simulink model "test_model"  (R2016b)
settings: Solver=VariableStepAuto  StartTime=0.0  StopTime=runtime  RelTol=1e-3
InitFcn:
  | clear mex
  | delete test_model_sfun.mexw64
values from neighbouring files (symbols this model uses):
  Delta_T = cell(1,4)    [modelParameters.m]
  F_D = 0    [modelParameters.m]
  g = 9.81    [modelParameters.m]
  Gamma_H = cell(1,4)    [modelParameters.m]
  have_motor_transient = 1    [modelParameters.m]
  height_controlled_o = (((Rm*If        + (((omega0_o * 2 * Rm * Kv * Kq      * Kd + 1)^2) - 1)/(4* Rm*Kv^2*Kq      * Kd))/Vb)*(Pmax - Pmin) + Pmin)    [modelParameters.m]
  i_0 = cell(1,4)    [modelParameters.m]
  If = 0.3836    [modelParameters.m]
  J = diag([ 0.0130 0.0140 0.0285 ])    [modelParameters.m]
  J_L = m_L/12*diag([y_L^2+z_L^2,x_L^2+z_L^2,x_L^2+y_L^2])    [modelParameters.m]
  J_r = cell(1,4)    [modelParameters.m]
  Jreq = 4.2012e-05    [modelParameters.m]
  Jxx = 0.0130    (= 0.013)    [modelParameters.m]
  Jyy = 0.0140    (= 0.014)    [modelParameters.m]
  Jzz = 0.0285    [modelParameters.m]
  K_d = cell(1,4)    [modelParameters.m]
  K_E = cell(1,4)    [modelParameters.m]
  K_H = cell(1,4)    [modelParameters.m]
  K_Q = cell(1,4)    [modelParameters.m]
  K_T = cell(1,4)    [modelParameters.m]
  K_V = cell(1,4)    [modelParameters.m]
  Kd = 1.4852e-07    [modelParameters.m]
  Ki_mahony = 0.001    [modelParameters.m]
  Kp_mahony = 0.4    [modelParameters.m]
  Kq = 96.3422    [modelParameters.m]
  Kt = 1.2007e-05    [modelParameters.m]
  Kv = 96.3422    [modelParameters.m]
  m = 1.216    [modelParameters.m]
  m_L = 0    [modelParameters.m]
  omega0_o = sqrt((m*g)/(4*Kt))    [modelParameters.m]
  omega1_o = sqrt((m*g)/(4*Kt))    [modelParameters.m]
  omega2_o = sqrt((m*g)/(4*Kt))    [modelParameters.m]
  omega3_o = sqrt((m*g)/(4*Kt))    [modelParameters.m]
  omega_0 = cell(1,4)    [modelParameters.m]
  p0 = 0    [modelParameters.m]
  p_0 = cell(1,4)    [modelParameters.m]
  p_max = cell(1,4)    [modelParameters.m]
  phi0 = 0    [modelParameters.m]
  pitch_o = 0    [modelParameters.m]
  pitchrate_o = 0    [modelParameters.m]
  Pmax = 1    [modelParameters.m]
  Pmin = 0    [modelParameters.m]
  psi0 = 0    [modelParameters.m]
  q0 = 0    [modelParameters.m]
  Q_D = 0    [modelParameters.m]
  r0 = 0    [modelParameters.m]
  R_m = cell(1,4)    [modelParameters.m]
  r_oc = [ 0 ; 0 ; 0 ]    [modelParameters.m]
  r_oL = [0; 0; 0]    [modelParameters.m]
  rhx = 0.16    [modelParameters.m]
  rhy = 0.16    [modelParameters.m]
  rhz = 0.03    [modelParameters.m]
  Rm = 0.235    [modelParameters.m]
  roll_o = 0    [modelParameters.m]
  rollrate_o = 0    [modelParameters.m]
  Tc = 0.04    [modelParameters.m]
  theta0 = 0    [modelParameters.m]
  Tq = 0.005    [modelParameters.m]
  u0 = 0    [modelParameters.m]
  v0 = 0    [modelParameters.m]
  Vb = 11.4    [modelParameters.m]
  w0 = 0    [modelParameters.m]
  x0 = 0    [modelParameters.m]
  x_controlled_o = 0    [modelParameters.m]
  x_o = 0    [modelParameters.m]
  x_vel_o = 0    [modelParameters.m]
  y0 = 0    [modelParameters.m]
  y_controlled_o = 0    [modelParameters.m]
  y_o = 0    [modelParameters.m]
  y_vel_o = 0    [modelParameters.m]
  yaw_controlled_o = 0    [modelParameters.m]
  yaw_o = 0    [modelParameters.m]
  yawrate_o = 0    [modelParameters.m]
  z0 = 0    [modelParameters.m]
  z_o = 0    [modelParameters.m]
  z_vel_o = 0    [modelParameters.m]
undefined symbols (not defined in the file or in its folder): Gamma_Omega, Gamma_T, Ki, Kp, r_h, slope, start, Ts, X0
libraries: simulink x16, Derivative x13, dsparch4 x3, vrlib x2
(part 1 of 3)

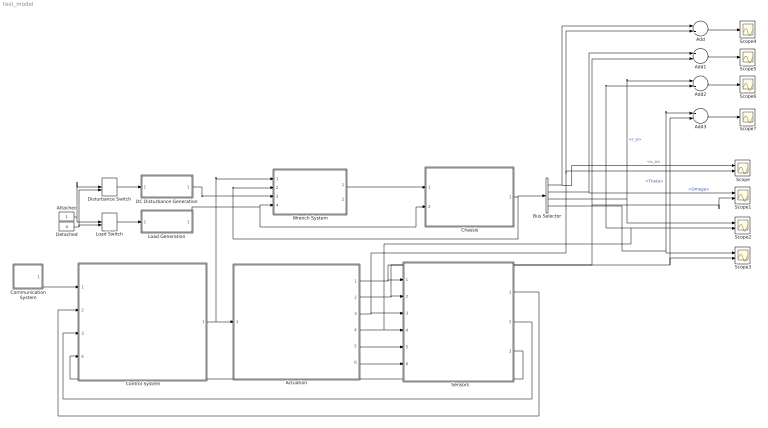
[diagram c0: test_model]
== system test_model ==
  "     Sensors   " : Subsystem
  Actuation : Subsystem
  Add{,1..3} (4 alike) : Sum  Inputs=+-
  Attached : Constant
  Bus Selector : BusSelector  OutputSignals=v_o,Omega,r_o,Theta
  Chassis : Subsystem
  Communication System : Subsystem
  Control System : Subsystem
  DC Disturbance Generation : Subsystem
  Detached : Constant  Value=0
  Disturbance Switch : ManualSwitch  CurrentSetting=0
  Load Generation : Subsystem
  Load Switch : ManualSwitch  CurrentSetting=0
  Scope{,1..3} (4 alike) : Scope  NumInputPorts=2
  Scope{4..7} (4 alike) : Scope
  Wrench System : Subsystem
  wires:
  Control System/1(P) -> Actuation/1(P), Wrench System/1(P)
  Communication System/1(setpoints) -> Control System/1(setpoints)
  Actuation/1(B_omega) -> Scope1/2, Add1/2, "     Sensors   "/1(B_Omega)
  Actuation/2(euler_angles) -> Scope3/2, Add3/2, "     Sensors   "/2(euler_angles)
  Actuation/3(B_vo) -> Scope/2, Add/2, "     Sensors   "/3(B_vo)
  Actuation/5(B_vo_dot) -> "     Sensors   "/5(B_vo_dot)
  Actuation/6(B_g) -> "     Sensors   "/6(B_g)
  "     Sensors   "/3(current_position) -> Control System/4(current_position)
  "     Sensors   "/2(euler_rates) -> Control System/3(euler_rates)
  "     Sensors   "/1(euler_angles_filtered) -> Control System/2(euler_angles_filtered)
  Wrench System/1(W) -> Chassis/1(W)
  Load Generation/1(Load) -> Chassis/2(Load), Wrench System/4(Load)
  DC Disturbance Generation/1(Disturbance) -> Wrench System/3(W_D)
  Attached/1 -> Load Switch/1, Disturbance Switch/1
  Detached/1 -> Load Switch/2, Disturbance Switch/2
  Load Switch/1 -> Load Generation/1(On/Off)
  Disturbance Switch/1 -> DC Disturbance Generation/1(On/Off)
  Chassis/1(Lambda) -> Wrench System/2(Lambda), Bus Selector/1
  Bus Selector/1 -> Add/1, Scope/1  "<v_o>"
  Bus Selector/2 -> Scope1/1, Add1/1  "<Omega>"
  Bus Selector/3 -> Scope2/1, Add2/1  "<r_o>"
  Actuation/4(E_ro) -> Add2/2, Scope2/2, "     Sensors   "/4(E_ro)
  Bus Selector/4 -> Add3/1, Scope3/1  "<Theta>"
  Add/1 -> Scope4/1
  Add3/1 -> Scope7/1
  Add2/1 -> Scope6/1
  Add1/1 -> Scope5/1

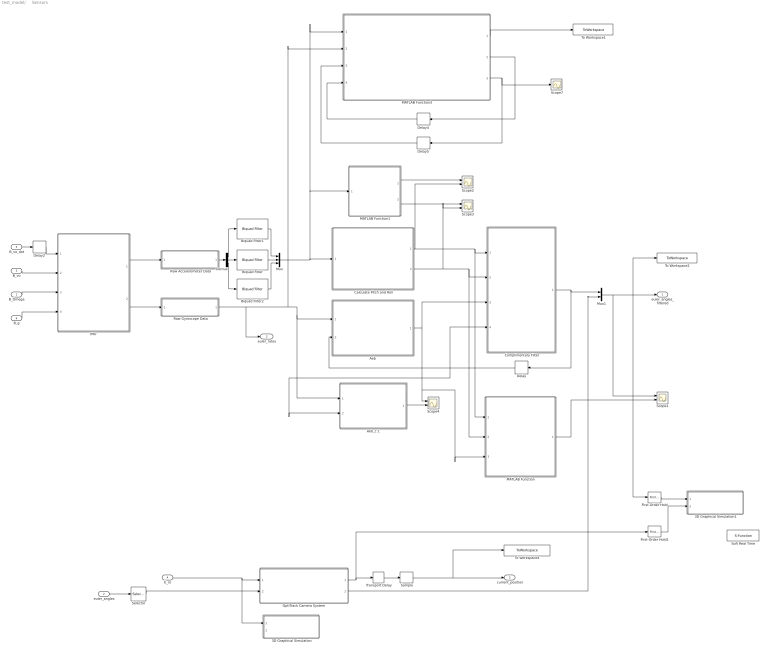
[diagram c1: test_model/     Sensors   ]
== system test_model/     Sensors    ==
  B_Omega : Inport
  euler_angles : Inport  Port=2
  B_vo : Inport  Port=3
  E_ro : Inport  Port=4
  B_vo_dot : Inport  Port=5
  B_g : Inport  Port=6
  3D Graphical Simulation : Subsystem  Commented=on
  3D Graphical Simulation1 : Subsystem  Commented=on
  "Aeb " : MATLAB Function  TreatAsAtomicUnit=on
  Aeb_c 1 : MATLAB Function  TreatAsAtomicUnit=on
  Biquad Filter : dsparch4/Biquad Filter  IIRFiltStruct=Direct form II  CoeffSource=Specify via dialog  BiQuadCoeffs=SOS_Matrix  a0Flag=Warning  IC=0  ICnum=0  ICden=0  InputProcessing=Columns as channels (frame based)  denAccumFracLength=30  denProdOutputFracLength=30  secondMemoryFracLength=15  roundingMode=Floor  overflowMode=off  ScaleValues=1  optimizeScaleValues=on  ScaleValueMode=Specify via input port (g)  scaleValueFracLength=14  FilterSource=Specify via dialog  FilterObject=BQF
  Biquad Filter1 : dsparch4/Biquad Filter  IIRFiltStruct=Direct form II  CoeffSource=Specify via dialog  BiQuadCoeffs=SOS_Matrix  a0Flag=Warning  IC=0  ICnum=0  ICden=0  InputProcessing=Columns as channels (frame based)  denAccumFracLength=30  denProdOutputFracLength=30  secondMemoryFracLength=15  roundingMode=Floor  overflowMode=off  ScaleValues=1  optimizeScaleValues=on  ScaleValueMode=Specify via input port (g)  scaleValueFracLength=14  FilterSource=Specify via dialog  FilterObject=BQF
  Biquad Filter2 : dsparch4/Biquad Filter  IIRFiltStruct=Direct form II  CoeffSource=Specify via dialog  BiQuadCoeffs=SOS_Matrix  a0Flag=Warning  IC=0  ICnum=0  ICden=0  InputProcessing=Columns as channels (frame based)  denAccumFracLength=30  denProdOutputFracLength=30  secondMemoryFracLength=15  roundingMode=Floor  overflowMode=off  ScaleValues=1  optimizeScaleValues=on  ScaleValueMode=Specify via input port (g)  scaleValueFracLength=14  FilterSource=Specify via dialog  FilterObject=BQF
  Calculate Pitch and Roll : MATLAB Function  TreatAsAtomicUnit=on
  Complimentary Filter : MATLAB Function  TreatAsAtomicUnit=on
  Delay : Delay  DelayLength=1  InitialCondition=0
  Delay2 : Delay  DelayLength=1  InitialCondition=0  SampleTime=Tq
  Delay4 : Delay  DelayLength=1  InitialCondition=0  SampleTime=Tq
  Delay5 : Delay  DelayLength=1  InitialCondition=[1, 0, 0, 0]  SampleTime=Tq
  Demux : Demux  Outputs=3
  First-Order Hold : simulink/Discrete/First-Order Hold  DisableCoverage=on  Ts=5e-3
  First-Order Hold1 : simulink/Discrete/First-Order Hold  DisableCoverage=on  Ts=5e-3
  "IMU " : Subsystem
  MATLAB Function : MATLAB Function  TreatAsAtomicUnit=on
  MATLAB Function1 : MATLAB Function  TreatAsAtomicUnit=on
  MATLAB Function3 : MATLAB Function  TreatAsAtomicUnit=on
  Mux : Mux  Inputs=3
  Mux1 : Mux  Inputs=2
  "OptiTrack Camera System " : Subsystem
  Raw Accelerometer Data : Subsystem  Variant=on
  Raw Gyroscope Data : Subsystem  Variant=on
  Sample : ZeroOrderHold  SampleTime=Tc
  Scope{1..4} (4 alike) : Scope  NumInputPorts=2
  Scope7 : Scope
  Selector : Selector  InputPortWidth=3  IndexOptions=Index vector (dialog)  Indices=[3]  OutputSizes=1
  Soft Real Time : S-Function  Commented=on  FunctionName=sfun_time  Parameters=x  SFunctionDeploymentMode=off  EnableBusSupport=off
  To Workspace1 : ToWorkspace  VariableName=mahony_reading  SaveFormat=Structure With Time  SampleTime=Tq
  To Workspace2 : ToWorkspace  VariableName=angle_IMU_reading  SaveFormat=Structure With Time  SampleTime=Tq
  To Workspace4 : ToWorkspace  VariableName=position_model  SaveFormat=Structure With Time  SampleTime=Tc
  Transport Delay : TransportDelay  DelayTime=6e-3
  euler_angles_filtered : Outport
  euler_rates : Outport  Port=2
  current_position : Outport  Port=3
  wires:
  "IMU "/1(accelerometer) -> Raw Accelerometer Data/1(raw_accel_model)
  "IMU "/2(gyroscope) -> Raw Gyroscope Data/1(raw_gyro_model)
  B_vo/1 -> "IMU "/2(B_vo)
  B_Omega/1 -> "IMU "/3(B_Omega)
  B_g/1 -> "IMU "/4(B_g)
  Calculate Pitch and Roll/2(accel_roll) -> Scope3/2, MATLAB Function/2(accel_roll), Complimentary Filter/2(accel_roll)
  Calculate Pitch and Roll/1(accel_pitch) -> MATLAB Function/1(accel_pitch), Complimentary Filter/1(accel_pitch), Scope2/2
  First-Order Hold/1 -> 3D Graphical Simulation1/1("Euler Angles ")
  E_ro/1 -> 3D Graphical Simulation/1(Displacement), "OptiTrack Camera System "/1(E_ro)
  First-Order Hold1/1 -> 3D Graphical Simulation1/2(Displacement)
  B_vo_dot/1 -> Delay2/1
  Delay2/1 -> "IMU "/1(B_vo_dot)
  "OptiTrack Camera System "/1(E_ro_camera) -> Transport Delay/1, First-Order Hold1/1
  Transport Delay/1 -> Sample/1
  Sample/1 -> To Workspace4/1, current_position/1
  Raw Gyroscope Data/1(raw_gyro) -> Aeb_c 1/1(gyro_reading), "Aeb "/1(gyro_reading), MATLAB Function3/2(gyroReadings), euler_rates/1
  Delay/1 -> Complimentary Filter/4(prev_euler_angles), Aeb_c 1/2(euler_angles_filtered), "Aeb "/2(euler_angles_filtered)
  Aeb_c 1/1(euler_rates_IMU) -> Scope4/2
  MATLAB Function1/1(accel_pitch) -> Scope2/1
  MATLAB Function1/2(accel_roll) -> Scope3/1
  "OptiTrack Camera System "/2(yaw_camera) -> Mux1/2
  MATLAB Function3/1(eulerAngles) -> To Workspace1/1
  MATLAB Function3/2(integralFeedback) -> Delay4/1
  Delay4/1 -> MATLAB Function3/4(integralFeedback_prev)
  MATLAB Function3/3(quaternions) -> Scope7/1, Delay5/1
  Delay5/1 -> MATLAB Function3/3(quaternions_prev)
  "Aeb "/1(euler_rates_IMU) -> MATLAB Function/3(euler_rates_gyro), Scope4/1, Complimentary Filter/3(euler_rates_gyro)
  Raw Accelerometer Data/1(raw_accel) -> Demux/1
  Demux/2 -> Biquad Filter/1
  Demux/1 -> Biquad Filter1/1
  Demux/3 -> Biquad Filter2/1
  Biquad Filter/1 -> Mux/2
  Biquad Filter1/1 -> Mux/1
  Biquad Filter2/1 -> Mux/3
  Mux/1 -> Calculate Pitch and Roll/1(accel_reading), MATLAB Function1/1(accel_reading), MATLAB Function3/1(accelReadings)
  Complimentary Filter/1(euler_angles_IMU) -> Mux1/1, Delay/1
  euler_angles/1 -> Selector/1
  Selector/1 -> "OptiTrack Camera System "/2(yaw)
  MATLAB Function/1(euler_angles_IMU) -> Scope1/2
  Mux1/1 -> Scope1/1, To Workspace2/1, First-Order Hold/1, euler_angles_filtered/1

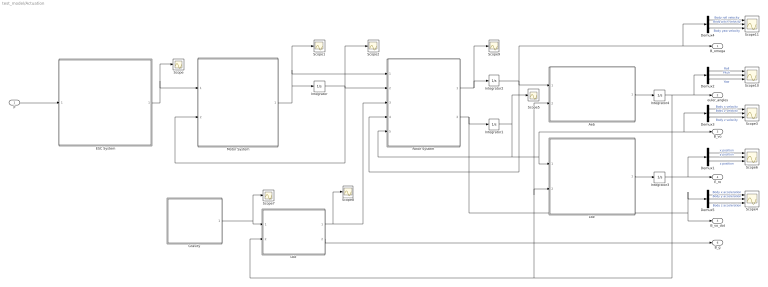
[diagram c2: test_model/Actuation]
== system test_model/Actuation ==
  P : Inport
  "Aeb " : MATLAB Function  TreatAsAtomicUnit=on
  Demux{1..5} (5 alike) : Demux  Outputs=3
  ESC System : MATLAB Function  TreatAsAtomicUnit=on
  "Gravity " : MATLAB Function  TreatAsAtomicUnit=on
  Integrator : Integrator  InitialCondition=[omega0_o, omega1_o, omega2_o, omega3_o]
  Integrator1 : Integrator  InitialCondition=[x_vel_o; y_vel_o; z_vel_o]
  Integrator2 : Integrator  InitialCondition=[rollrate_o; pitchrate_o; yawrate_o]
  Integrator3 : Integrator  InitialCondition=[x_o; y_o; z_o]
  Integrator4 : Integrator  InitialCondition=[roll_o; pitch_o; yaw_o]  ContinuousStateAttributes=['phi' 'theta' 'psi']
  "Lbe " : MATLAB Function  TreatAsAtomicUnit=on
  "Lbe " : MATLAB Function  TreatAsAtomicUnit=on
  Motor System : MATLAB Function  TreatAsAtomicUnit=on
  "Rotor System " : MATLAB Function  TreatAsAtomicUnit=on
  Scope{,1..2,5,7..9} (7 alike) : Scope
  Scope{3..4,6,10..11} (5 alike) : Scope  NumInputPorts=3
  B_omega : Outport
  euler_angles : Outport  Port=2
  B_vo : Outport  Port=3
  E_ro : Outport  Port=4
  B_vo_dot : Outport  Port=5
  B_g : Outport  Port=6
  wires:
  ESC System/1(Vb_eff) -> Scope/1, Motor System/1(Vb_eff)
  Motor System/1(w_dot) -> Integrator/1, Scope1/1, "Rotor System "/1(w_dot)
  "Rotor System "/1(B_omega_dot) -> Scope9/1, Integrator2/1
  Integrator2/1 -> "Rotor System "/4(B_omega), B_omega/1, Demux4/1, "Aeb "/1(B_omega)
  "Aeb "/1(euler_rates) -> Integrator4/1
  "Lbe "/1(E_ro) -> Integrator3/1
  Integrator3/1 -> Demux1/1, E_ro/1
  "Lbe "/1(B_Fg) -> Scope8/1, "Rotor System "/3(B_Fg)
  "Lbe "/2(B_g) -> B_g/1
  Demux1/2 -> Scope6/2  "y position"
  Demux1/1 -> Scope6/1  "x position"
  Demux1/3 -> Scope6/3  "z position"
  Demux2/2 -> Scope10/2  "Pitch"
  Demux2/1 -> Scope10/1  "Roll"
  Demux2/3 -> Scope10/3  "Yaw"
  Demux4/2 -> Scope11/2  "Body pitch velocity"
  Demux4/1 -> Scope11/1  "Body roll velocity"
  Demux4/3 -> Scope11/3  "Body yaw velocity"
  Demux3/2 -> Scope3/2  "Body y velocity"
  Demux3/1 -> Scope3/1  "Body x velocity"
  Demux3/3 -> Scope3/3  "Body z velocity"
  Demux5/2 -> Scope4/2  "Body y acceleration"
  Demux5/1 -> Scope4/1  "Body x acceleration"
  Demux5/3 -> Scope4/3  "Body z acceleration"
  Integrator1/1 -> Scope5/1, "Rotor System "/5(B_vo), "Lbe "/1(B_vo), Demux3/1, B_vo/1
  "Rotor System "/2(B_vo_dot) -> Demux5/1, B_vo_dot/1, Integrator1/1
  Integrator4/1 -> euler_angles/1, Demux2/1, "Lbe "/2(euler_angles), "Aeb "/2(euler_angles), "Lbe "/2(euler_angles)
  P/1 -> ESC System/1(P)
  "Gravity "/1(E_Fg) -> Scope7/1, "Lbe "/1(E_Fg)
  Integrator/1 -> Motor System/2(w), "Rotor System "/2(w), Scope2/1

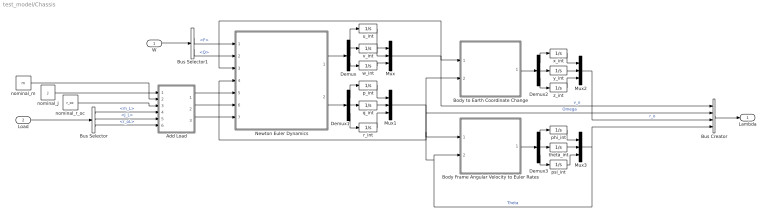
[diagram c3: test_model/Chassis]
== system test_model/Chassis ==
  W : Inport
  Load : Inport  Port=2
  Add Load : Subsystem
  Body Frame Angular Velocity to Euler Rates : MATLAB Function  TreatAsAtomicUnit=on
  Body to Earth Coordinate Change : MATLAB Function  TreatAsAtomicUnit=on
  Bus Creator : BusCreator  Inputs=4
  Bus Selector : BusSelector  OutputSignals=m_L,J_L,r_oL
  Bus Selector1 : BusSelector  OutputSignals=F,Q
  Demux{,1..3} (4 alike) : Demux  Outputs=3
  Mux{,1..3} (4 alike) : Mux  Inputs=3
  Newton Euler Dynamics : Subsystem
  nominal_J : Constant  Value=J
  nominal_m : Constant  Value=m
  nominal_r_oc : Constant  Value=r_oc
  p_int : Integrator  InitialCondition=p0  ContinuousStateAttributes='p'
  phi_int : Integrator  InitialCondition=phi0  ContinuousStateAttributes='phi'
  psi_int : Integrator  InitialCondition=psi0  ContinuousStateAttributes='psi'
  q_int : Integrator  InitialCondition=q0  ContinuousStateAttributes='q'
  r_int : Integrator  InitialCondition=r0  ContinuousStateAttributes='r'
  theta_int : Integrator  InitialCondition=theta0  ContinuousStateAttributes='theta'
  u_int : Integrator  InitialCondition=u0  ContinuousStateAttributes='u'
  v_int : Integrator  InitialCondition=v0  ContinuousStateAttributes='v'
  w_int : Integrator  InitialCondition=w0  ContinuousStateAttributes='w'
  x_int : Integrator  InitialCondition=x0  ContinuousStateAttributes='x'
  y_int : Integrator  InitialCondition=y0  ContinuousStateAttributes='y'
  z_int : Integrator  InitialCondition=z0  ContinuousStateAttributes='z'
  Lambda : Outport
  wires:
  nominal_J/1 -> Add Load/2(J_0)
  Bus Selector/3 -> Add Load/6(r_ol)  "<r_oL>"
  Bus Selector/2 -> Add Load/5(J_l)  "<J_L>"
  Bus Selector/1 -> Add Load/4(m_l)  "<m_L>"
  Add Load/3(r_oc) -> Newton Euler Dynamics/7(r_oc)
  Add Load/2(J) -> Newton Euler Dynamics/6(J)
  Add Load/1(m) -> Newton Euler Dynamics/5(m)
  W/1 -> Bus Selector1/1
  Bus Selector1/2 -> Newton Euler Dynamics/2(Q)  "<Q>"
  Bus Selector1/1 -> Newton Euler Dynamics/1(F)  "<F>"
  Body Frame Angular Velocity to Euler Rates/1(dot_Theta) -> Demux3/1
  Demux3/3 -> psi_int/1
  Demux3/2 -> theta_int/1
  Demux3/1 -> phi_int/1
  psi_int/1 -> Mux3/3
  theta_int/1 -> Mux3/2
  phi_int/1 -> Mux3/1
  Body to Earth Coordinate Change/1(x_E) -> Demux2/1
  Demux2/3 -> z_int/1
  Demux2/2 -> y_int/1
  Demux2/1 -> x_int/1
  z_int/1 -> Mux2/3
  y_int/1 -> Mux2/2
  x_int/1 -> Mux2/1
  Newton Euler Dynamics/2(dOmega) -> Demux1/1
  Demux1/3 -> r_int/1
  Demux1/2 -> q_int/1
  Demux1/1 -> p_int/1
  r_int/1 -> Mux1/3
  q_int/1 -> Mux1/2
  p_int/1 -> Mux1/1
  Newton Euler Dynamics/1(dv) -> Demux/1
  Demux/3 -> w_int/1
  Demux/2 -> v_int/1
  Demux/1 -> u_int/1
  w_int/1 -> Mux/3
  v_int/1 -> Mux/2
  u_int/1 -> Mux/1
  Bus Creator/1 -> Lambda/1
  Mux3/1 -> Body to Earth Coordinate Change/2(Theta), Body Frame Angular Velocity to Euler Rates/2(Theta), Bus Creator/4  "Theta"
  Mux2/1 -> Bus Creator/3  "r_o"
  Mux1/1 -> Body Frame Angular Velocity to Euler Rates/1(Omega_B), Newton Euler Dynamics/4(Omega), Bus Creator/2  "Omega"
  Mux/1 -> Bus Creator/1, Body to Earth Coordinate Change/1(x_B), Newton Euler Dynamics/3(v)  "v_o"
  nominal_m/1 -> Add Load/1(m_0)
  nominal_r_oc/1 -> Add Load/3(r_oc_0)
  Load/1 -> Bus Selector/1

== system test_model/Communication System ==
  Step : Step  Before=[0; 0; 0; 0]  After=[1; 0; 0; 0]  SampleTime=Tq
  setpoints : Outport
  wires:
  Step/1 -> setpoints/1

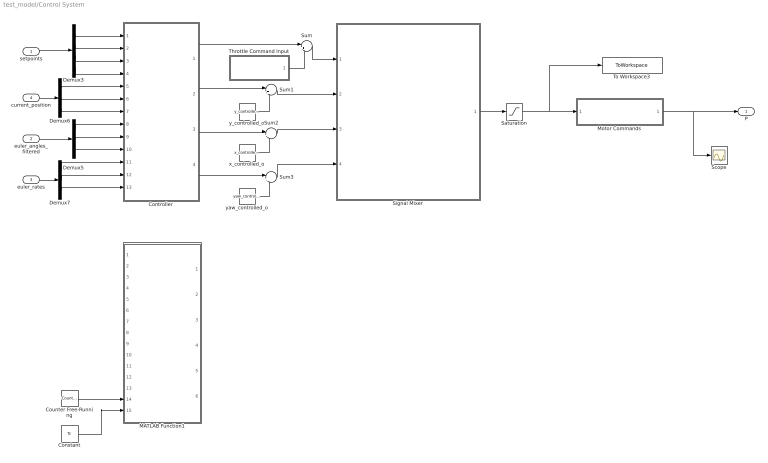
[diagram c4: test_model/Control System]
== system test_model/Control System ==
  setpoints : Inport
  euler_angles_filtered : Inport  Port=2
  euler_rates : Inport  Port=3
  current_position : Inport  Port=4
  Constant : Constant  Value=Tc  SampleTime=Tc
  Controller : Subsystem
  Counter Free-Running : simulink/Sources/Counter Free-Running  NumBits=32  tsamp=Tc
  Demux3 : Demux
  Demux5 : Demux  Outputs=3
  Demux6 : Demux  Outputs=3
  Demux7 : Demux  Outputs=3
  MATLAB Function1 : MATLAB Function  Commented=on  TreatAsAtomicUnit=on  SystemSampleTime=Tq
  Motor Commands : Subsystem  Variant=on
  Saturation : Saturate  UpperLimit=Pmax*ones(4,1)  LowerLimit=Pmin*ones(4,1)
  Scope : Scope
  Signal Mixer : MATLAB Function  TreatAsAtomicUnit=on
  Sum{,1..3} (4 alike) : Sum  Inputs=|++
  Throttle Command Input : Subsystem  Variant=on
  To Workspace3 : ToWorkspace  VariableName=motorCommands  SaveFormat=Structure With Time  SampleTime=Tq
  x_controlled_o : Constant  Value=x_controlled_o
  y_controlled_o : Constant  Value=y_controlled_o
  yaw_controlled_o : Constant  Value=yaw_controlled_o
  P : Outport
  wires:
  y_controlled_o/1 -> Sum1/2
  x_controlled_o/1 -> Sum2/2
  yaw_controlled_o/1 -> Sum3/2
  Signal Mixer/1(P) -> Saturation/1
  Counter Free-Running/1 -> MATLAB Function1/14(vrpn_id)
  Constant/1 -> MATLAB Function1/15(Tc)
  Sum1/1 -> Signal Mixer/2(y_controlled)
  Sum2/1 -> Signal Mixer/3(x_controlled)
  Sum3/1 -> Signal Mixer/4(yaw_controlled)
  Motor Commands/1(z_command) -> P/1, Scope/1
  Saturation/1 -> To Workspace3/1, Motor Commands/1(z_command_model)
  setpoints/1 -> Demux3/1
  current_position/1 -> Demux6/1
  euler_angles_filtered/1 -> Demux5/1
  euler_rates/1 -> Demux7/1
  Demux3/1 -> Controller/1(x_setpoint)
  Demux3/2 -> Controller/2(y_setpoint)
  Demux3/3 -> Controller/3(z_setpoint)
  Demux3/4 -> Controller/4(yaw_setpoint)
  Demux6/1 -> Controller/5(x_position)
  Demux6/2 -> Controller/6(y_position)
  Demux6/3 -> Controller/7(z_position)
  Demux5/1 -> Controller/8(roll)
  Demux5/2 -> Controller/9(pitch)
  Demux5/3 -> Controller/10(yaw)
  Demux7/1 -> Controller/11(roll_rate)
  Demux7/2 -> Controller/12(pitch_rate)
  Demux7/3 -> Controller/13(yaw_rate)
  Controller/1(height_controlled) -> Sum/1
  Controller/2(y_controlled) -> Sum1/1
  Controller/3(x_controlled) -> Sum2/1
  Controller/4(yaw_controlled) -> Sum3/1
  Throttle Command Input/1(z_command) -> Sum/2
  Sum/1 -> Signal Mixer/1(height_controlled)

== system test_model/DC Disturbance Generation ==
  On/Off : Inport
  Bus Creator2 : BusCreator  Inputs=2
  Compare To Zero : Subsystem
  F_D : Constant  Value=F_D
  Product : Product
  Product1 : Product
  Q_D : Constant  Value=Q_D
  Disturbance : Outport
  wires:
  Compare To Zero/1(y) -> Product/2, Product1/2
  On/Off/1 -> Compare To Zero/1(u)
  Q_D/1 -> Product1/1  "Q_D"
  F_D/1 -> Product/1  "F_D"
  Bus Creator2/1 -> Disturbance/1
  Product1/1 -> Bus Creator2/2  "Q_D"
  Product/1 -> Bus Creator2/1  "F_D"

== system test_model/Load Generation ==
  On/Off : Inport
  Bus Creator1 : BusCreator  Inputs=3
  Compare To Zero : Subsystem
  J_L : Constant  Value=J_L
  Product : Product
  Product1 : Product
  Product2 : Product
  m_L : Constant  Value=m_L
  r_oL : Constant  Value=r_oL
  Load : Outport
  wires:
  Compare To Zero/1(y) -> Product/2, Product1/2, Product2/2
  On/Off/1 -> Compare To Zero/1(u)
  J_L/1 -> Product1/1  "J_L"
  r_oL/1 -> Product2/1  "r_oL"
  m_L/1 -> Product/1  "m_L"
  Bus Creator1/1 -> Load/1
  Product2/1 -> Bus Creator1/3  "r_oL"
  Product1/1 -> Bus Creator1/2  "J_L"
  Product/1 -> Bus Creator1/1  "m_L"

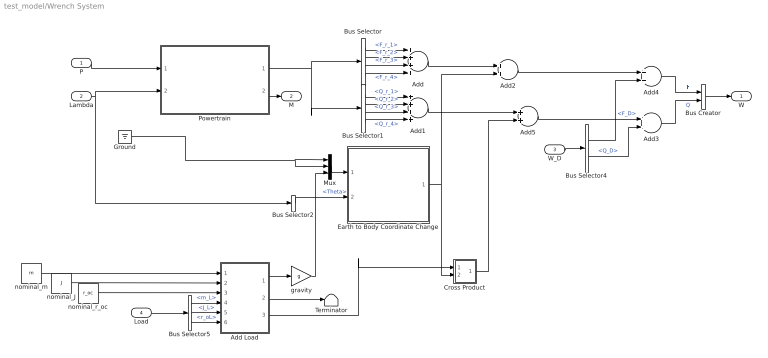
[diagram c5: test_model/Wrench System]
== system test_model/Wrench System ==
  P : Inport
  Lambda : Inport  Port=2
  W_D : Inport  Port=3
  Load : Inport  Port=4
  Add : Sum  Inputs=++++
  Add Load : Subsystem
  Add1 : Sum  Inputs=++++
  Add{2..5} (4 alike) : Sum
  Bus Creator : BusCreator  Inputs=2
  Bus Selector : BusSelector  OutputSignals=F_r_1,F_r_2,F_r_3,F_r_4
  Bus Selector1 : BusSelector  OutputSignals=Q_r_1,Q_r_2,Q_r_3,Q_r_4
  Bus Selector2 : BusSelector  OutputSignals=Theta
  Bus Selector4 : BusSelector  OutputSignals=F_D,Q_D
  Bus Selector5 : BusSelector  OutputSignals=m_L,J_L,r_oL
  Cross Product : Subsystem
  Earth to Body Coordinate Change : MATLAB Function  TreatAsAtomicUnit=on
  Ground : Ground
  Mux : Mux  Inputs=3
  Powertrain : Subsystem
  Terminator : Terminator
  gravity : Gain  Gain=g
  nominal_J : Constant  Value=J
  nominal_m : Constant  Value=m
  nominal_r_oc : Constant  Value=r_oc
  W : Outport
  M : Outport  Port=2
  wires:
  Add Load/2(J) -> Terminator/1
  Cross Product/1(y) -> Add5/2
  Add1/1 -> Add5/1
  Add5/1 -> Add3/1
  gravity/1 -> Mux/3
  Add Load/3(r_oc) -> Cross Product/1(a)
  Add Load/1(m) -> gravity/1
  Load/1 -> Bus Selector5/1
  Bus Selector5/3 -> Add Load/6(r_ol)  "<r_oL>"
  Bus Selector5/2 -> Add Load/5(J_l)  "<J_L>"
  Bus Selector5/1 -> Add Load/4(m_l)  "<m_L>"
  nominal_r_oc/1 -> Add Load/3(r_oc_0)
  nominal_J/1 -> Add Load/2(J_0)
  nominal_m/1 -> Add Load/1(m_0)
  Mux/1 -> Earth to Body Coordinate Change/1(x_E)
  Ground/1 -> Mux/2, Mux/1
  Powertrain/2(M) -> M/1
  W_D/1 -> Bus Selector4/1
  Bus Creator/1 -> W/1
  Add3/1 -> Bus Creator/2  "Q"
  Add4/1 -> Bus Creator/1  "F"
  Bus Selector4/2 -> Add3/2  "<Q_D>"
  Bus Selector4/1 -> Add4/2  "<F_D>"
  Add2/1 -> Add4/1
  Earth to Body Coordinate Change/1(x_B) -> Cross Product/2(b), Add2/2
  Add/1 -> Add2/1
  Bus Selector2/1 -> Earth to Body Coordinate Change/2(Theta)  "<Theta>"
  Powertrain/1(W_r) -> Bus Selector1/1, Bus Selector/1
  Bus Selector/1 -> Add/1  "<F_r_1>"
  Bus Selector/2 -> Add/2  "<F_r_2>"
  Bus Selector/3 -> Add/3  "<F_r_3>"
  Bus Selector/4 -> Add/4  "<F_r_4>"
  Bus Selector1/1 -> Add1/1  "<Q_r_1>"
  Bus Selector1/2 -> Add1/2  "<Q_r_2>"
  Bus Selector1/3 -> Add1/3  "<Q_r_3>"
  Bus Selector1/4 -> Add1/4  "<Q_r_4>"
  P/1 -> Powertrain/1(P)
  Lambda/1 -> Bus Selector2/1, Powertrain/2(Lambda)

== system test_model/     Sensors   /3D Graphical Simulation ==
  Displacement : Inport
  Euler Angles : Inport  Port=2
  Bus Creator : BusCreator  Inputs=3
  Bus Creator1 : BusCreator  Inputs=3
  Bus Creator2 : BusCreator  Inputs=3
  Bus Selector : BusSelector  OutputSignals=phi,theta,psi
  Demux : Demux  Outputs=3
  Demux1 : Demux  Outputs=3
  Gain : Gain  Gain=-1
  Gain1 : Gain  Gain=eye(3)*1  Multiplication=Matrix(K*u)
  Gain2 : Gain  Gain=-1
  MATLAB Function : MATLAB Function  TreatAsAtomicUnit=on
  Rate Transition : RateTransition  OutPortSampleTime=0.06
  Rate Transition1 : RateTransition  OutPortSampleTime=0.06
  VR Sink : vrlib/VR Sink  InstantiateOnLoad=on  SampleTime=-1  ViewEnable=on  RemoteChange=off  RemoteView=off  FieldsWritten=Helicopter.rotation.4.1.1.double#Helicopter.translation.3.1.1.double  WorldFileName=quadrotor_world_ucart.wrl  AutoView=on  VideoDimensions=[]  AllowVariableSize=off
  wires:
  Displacement/1 -> Demux/1
  Bus Creator2/1 -> Bus Selector/1
  Demux/1 -> Bus Creator1/3
  Gain/1 -> Bus Creator1/2
  Gain2/1 -> Bus Creator1/1
  Rate Transition1/1 -> VR Sink/2
  Rate Transition/1 -> VR Sink/1
  Demux/3 -> Gain/1
  Demux/2 -> Gain2/1
  Bus Creator1/1 -> Gain1/1
  Bus Selector/1 -> Bus Creator/3  "<phi>"
  Bus Selector/3 -> Bus Creator/2  "<psi>"
  Bus Selector/2 -> Bus Creator/1  "<theta>"
  Gain1/1 -> Rate Transition1/1
  Demux1/3 -> Bus Creator2/3  "psi"
  Demux1/2 -> Bus Creator2/2  "theta"
  Demux1/1 -> Bus Creator2/1  "phi"
  Euler Angles/1 -> Demux1/1
  Bus Creator/1 -> MATLAB Function/1(u)
  MATLAB Function/1(y) -> Rate Transition/1

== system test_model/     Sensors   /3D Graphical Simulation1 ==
  "Euler Angles " : Inport
  Displacement : Inport  Port=2
  Bus Creator : BusCreator  Inputs=3
  Bus Creator1 : BusCreator  Inputs=3
  Bus Creator2 : BusCreator  Inputs=3
  Bus Selector : BusSelector  OutputSignals=phi,theta,psi
  Demux : Demux  Outputs=3
  Demux1 : Demux  Outputs=3
  Gain : Gain  Gain=-1
  Gain1 : Gain  Gain=eye(3)*1  Multiplication=Matrix(K*u)
  Gain2 : Gain  Gain=-1
  MATLAB Function : MATLAB Function  TreatAsAtomicUnit=on
  Rate Transition : RateTransition  OutPortSampleTime=0.06
  Rate Transition1 : RateTransition  OutPortSampleTime=0.06
  VR Sink : vrlib/VR Sink  InstantiateOnLoad=on  SampleTime=-1  ViewEnable=on  RemoteChange=off  RemoteView=off  FieldsWritten=Helicopter.rotation.4.1.1.double#Helicopter.translation.3.1.1.double  WorldFileName=quadrotor_world_ucart.wrl  AutoView=on  VideoDimensions=[]  AllowVariableSize=off
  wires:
  Bus Creator2/1 -> Bus Selector/1
  Demux/1 -> Bus Creator1/3
  Gain/1 -> Bus Creator1/2
  Gain2/1 -> Bus Creator1/1
  Rate Transition1/1 -> VR Sink/2
  Rate Transition/1 -> VR Sink/1
  Demux/3 -> Gain/1
  Demux/2 -> Gain2/1
  Bus Creator1/1 -> Gain1/1
  Bus Selector/1 -> Bus Creator/3  "<phi>"
  Bus Selector/3 -> Bus Creator/2  "<psi>"
  Bus Selector/2 -> Bus Creator/1  "<theta>"
  Gain1/1 -> Rate Transition1/1
  Demux1/3 -> Bus Creator2/3  "psi"
  Demux1/2 -> Bus Creator2/2  "theta"
  Demux1/1 -> Bus Creator2/1  "phi"
  Bus Creator/1 -> MATLAB Function/1(u)
  MATLAB Function/1(y) -> Rate Transition/1
  Displacement/1 -> Demux/1
  "Euler Angles "/1 -> Demux1/1

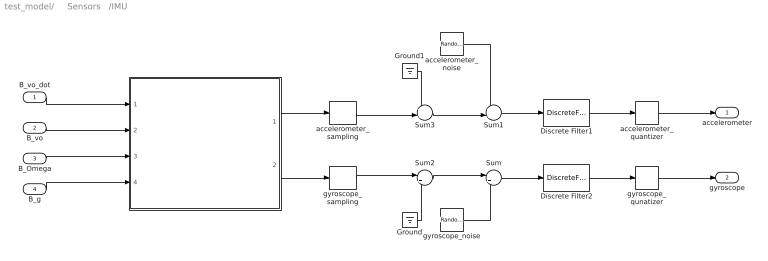
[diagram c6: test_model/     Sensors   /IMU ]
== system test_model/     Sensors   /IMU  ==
  B_vo_dot : Inport
  B_vo : Inport  Port=2
  B_Omega : Inport  Port=3
  B_g : Inport  Port=4
  " " : MATLAB Function  TreatAsAtomicUnit=on
  Discrete Filter1 : DiscreteFilter  Numerator=[0 0.749]  Denominator=[1 -0.251]  InitialStates=[0, 0, -1]  SampleTime=Tq
  Discrete Filter2 : DiscreteFilter  Numerator=[0 0.7327]  Denominator=[1 -0.2673]  SampleTime=Tq
  Ground : Ground
  Ground1 : Ground
  Sum : Sum  Inputs=|++
  Sum1 : Sum  Inputs=++|
  Sum2 : Sum  Inputs=|++
  Sum3 : Sum  Inputs=++|
  accelerometer_noise : RandomNumber  Mean=zeros(3,1)  Variance=[ 3e-7 ; 3.3e-7 ; 7.2e-7 ]  Seed=[0,1,2]  SampleTime=Tq
  accelerometer_quantizer : Quantizer  QuantizationInterval=2.4400e-04
  accelerometer_sampling : ZeroOrderHold  SampleTime=Tq
  gyroscope_noise : RandomNumber  Mean=zeros(3,1)  Variance=[ 2.2e-8 ; 1.1e-7 ; 2.4e-8 ]  Seed=[0,1,2]  SampleTime=Tq
  gyroscope_qunatizer : Quantizer  QuantizationInterval=1.1e-3
  gyroscope_sampling : ZeroOrderHold  SampleTime=Tq
  accelerometer : Outport
  gyroscope : Outport  Port=2
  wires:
  accelerometer_noise/1 -> Sum1/1
  Sum2/1 -> Sum/1
  Sum3/1 -> Sum1/2
  gyroscope_noise/1 -> Sum/2
  gyroscope_sampling/1 -> Sum2/1
  accelerometer_sampling/1 -> Sum3/2
  Ground/1 -> Sum2/2
  Ground1/1 -> Sum3/1
  B_vo_dot/1 -> " "/1(B_vo_dot)
  B_vo/1 -> " "/2(B_vo)
  B_Omega/1 -> " "/3(B_Omega)
  B_g/1 -> " "/4(B_g)
  " "/2(gyroReading) -> gyroscope_sampling/1
  " "/1(accelReading) -> accelerometer_sampling/1
  Sum1/1 -> Discrete Filter1/1
  Sum/1 -> Discrete Filter2/1
  accelerometer_quantizer/1 -> accelerometer/1
  gyroscope_qunatizer/1 -> gyroscope/1
  Discrete Filter1/1 -> accelerometer_quantizer/1
  Discrete Filter2/1 -> gyroscope_qunatizer/1

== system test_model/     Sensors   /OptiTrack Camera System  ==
  E_ro : Inport
  yaw : Inport  Port=2
  E_ro_noise : RandomNumber  Mean=zeros(3,1)  Variance=[ 7.9664e-10 ; 1.1928e-10 ; 5.0636e-10 ]  Seed=[0,1,2]  SampleTime=Tc
  E_ro_quantizer : Quantizer  QuantizationInterval=2.4400e-04
  E_ro_sampling : ZeroOrderHold  SampleTime=Tc
  Ground1 : Ground
  Ground2 : Ground
  Sum1 : Sum  Inputs=++|
  Sum3 : Sum  Inputs=++|
  Sum4 : Sum  Inputs=|++
  Sum6 : Sum  Inputs=|++
  yaw_noise : RandomNumber  Variance=1.0783e-9  SampleTime=Tq
  yaw_quantizer : Quantizer  QuantizationInterval=1.1e-3
  yaw_sampling : ZeroOrderHold  SampleTime=Tq
  E_ro_camera : Outport
  yaw_camera : Outport  Port=2
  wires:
  E_ro_noise/1 -> Sum1/1
  Sum3/1 -> Sum1/2
  Sum1/1 -> E_ro_quantizer/1
  E_ro_sampling/1 -> Sum3/2
  Ground1/1 -> Sum3/1
  Sum4/1 -> yaw_quantizer/1
  Sum6/1 -> Sum4/1
  yaw_noise/1 -> Sum4/2
  yaw_sampling/1 -> Sum6/1
  Ground2/1 -> Sum6/2
  yaw/1 -> yaw_sampling/1
  E_ro/1 -> E_ro_sampling/1
  E_ro_quantizer/1 -> E_ro_camera/1
  yaw_quantizer/1 -> yaw_camera/1

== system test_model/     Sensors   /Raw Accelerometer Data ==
  note: 1) Add Subsystem or Model blocks as valid variant choices. 2) You cannot connect blocks at this level. At simulation, connectivity is automatically determined, based on the active variant and port name matching.
  raw_accel_model : Inport
  Feedback : Subsystem  VariantControl=logAnalysisToggle==0
  "Raw Accelerometer Data " : Subsystem  VariantControl=logAnalysisToggle==1
  raw_accel : Outport

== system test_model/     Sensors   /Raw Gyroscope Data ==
  note: 1) Add Subsystem or Model blocks as valid variant choices. 2) You cannot connect blocks at this level. At simulation, connectivity is automatically determined, based on the active variant and port name matching.
  raw_gyro_model : Inport
  Feedback : Subsystem  VariantControl=logAnalysisToggle==0
  "Raw Gyroscope Data " : Subsystem  VariantControl=logAnalysisToggle==1
  raw_gyro : Outport

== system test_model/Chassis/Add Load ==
  m_0 : Inport
  J_0 : Inport  Port=2
  r_oc_0 : Inport  Port=3
  m_l : Inport  Port=4
  J_l : Inport  Port=5
  r_ol : Inport  Port=6
  Add Load to Quadrotor : MATLAB Function  TreatAsAtomicUnit=on
  m : Outport
  J : Outport  Port=2
  r_oc : Outport  Port=3
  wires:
  r_ol/1 -> Add Load to Quadrotor/6(r_ol)
  Add Load to Quadrotor/3(r_oc) -> r_oc/1
  J_l/1 -> Add Load to Quadrotor/5(J_l)
  m_l/1 -> Add Load to Quadrotor/4(m_l)
  Add Load to Quadrotor/2(J) -> J/1
  r_oc_0/1 -> Add Load to Quadrotor/3(r_oc_0)
  J_0/1 -> Add Load to Quadrotor/2(J_0)
  Add Load to Quadrotor/1(m) -> m/1
  m_0/1 -> Add Load to Quadrotor/1(m_0)

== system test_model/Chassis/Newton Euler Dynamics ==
  F : Inport
  Q : Inport  Port=2
  v : Inport  Port=3
  Omega : Inport  Port=4
  m : Inport  Port=5
  J : Inport  Port=6
  r_oc : Inport  Port=7
  Newton-Euler Rigid Body Dynamics : MATLAB Function  TreatAsAtomicUnit=on
  dv : Outport
  dOmega : Outport  Port=2
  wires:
  m/1 -> Newton-Euler Rigid Body Dynamics/5(m)
  J/1 -> Newton-Euler Rigid Body Dynamics/6(J)
  r_oc/1 -> Newton-Euler Rigid Body Dynamics/7(r_oc)
  F/1 -> Newton-Euler Rigid Body Dynamics/1(F)
  Q/1 -> Newton-Euler Rigid Body Dynamics/2(Q)
  v/1 -> Newton-Euler Rigid Body Dynamics/3(v)
  Omega/1 -> Newton-Euler Rigid Body Dynamics/4(Omega)
  Newton-Euler Rigid Body Dynamics/1(dv) -> dv/1
  Newton-Euler Rigid Body Dynamics/2(dOmega) -> dOmega/1

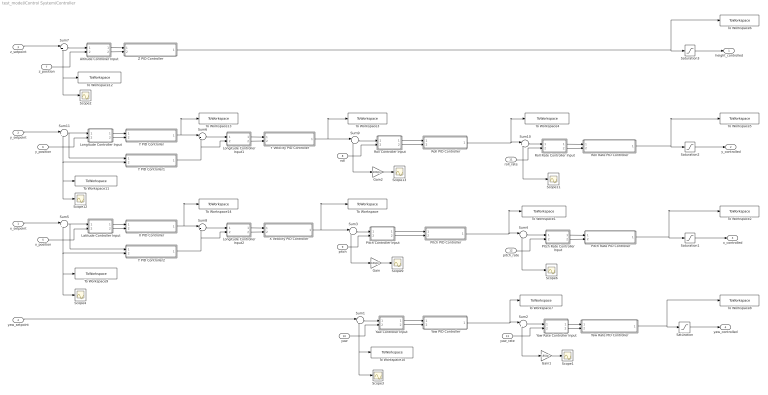
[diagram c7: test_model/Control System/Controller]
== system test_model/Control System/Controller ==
  x_setpoint : Inport
  y_setpoint : Inport  Port=2
  z_setpoint : Inport  Port=3
  yaw_setpoint : Inport  Port=4
  x_position : Inport  Port=5
  y_position : Inport  Port=6
  z_position : Inport  Port=7
  roll : Inport  Port=8
  pitch : Inport  Port=9
  yaw : Inport  Port=10
  roll_rate : Inport  Port=11
  pitch_rate : Inport  Port=12
  yaw_rate : Inport  Port=13
  Altitude Controller Input : Subsystem  Variant=on
  Gain : Gain  Gain=180/pi
  Gain1 : Gain  Gain=180/pi
  Gain2 : Gain  Gain=180/pi
  Latitude Controller Input : Subsystem  Variant=on
  Longitude Controller Input : Subsystem  Variant=on
  Longitude Controller Input1 : Subsystem  Variant=on
  Longitude Controller Input2 : Subsystem  Variant=on
  Pitch Controller Input : Subsystem  Variant=on
  Pitch PID Controller : Subsystem
  Pitch Rate Controller Input : Subsystem  Variant=on
  Pitch Rate PID Controller : Subsystem
  Roll Controller Input : Subsystem  Variant=on
  Roll PID Controller : Subsystem
  Roll Rate Controller Input : Subsystem  Variant=on
  Roll Rate PID Controller : Subsystem
  Saturation{,1..3} (4 alike) : Saturate  UpperLimit=20000  LowerLimit=-20000
  Scope{1..4,6,9,11..13} (9 alike) : Scope
  Sum{1..11} (11 alike) : Sum  Inputs=|+-
  To Workspace : ToWorkspace  VariableName=pitch_setpoint_model  SaveFormat=Structure With Time  SampleTime=-1
  To Workspace1 : ToWorkspace  VariableName=pitchrate_setpoint_model  SaveFormat=Structure With Time  SampleTime=Tq
  To Workspace10 : ToWorkspace  VariableName=yaw_value_model  SaveFormat=Structure With Time  SampleTime=Tc
  To Workspace11 : ToWorkspace  VariableName=y_position_model  SaveFormat=Structure With Time  SampleTime=Tc
  To Workspace12 : ToWorkspace  VariableName=z_position_model  SaveFormat=Structure With Time  SampleTime=Tc
  To Workspace13 : ToWorkspace  VariableName=y_vel_setpoint_model  SaveFormat=Structure With Time  SampleTime=Tc
  To Workspace14 : ToWorkspace  VariableName=x_vel_setpoint_model  SaveFormat=Structure With Time  SampleTime=Tc
  To Workspace2 : ToWorkspace  VariableName=x_command_model  SaveFormat=Structure With Time  SampleTime=Tq
  To Workspace3 : ToWorkspace  VariableName=roll_setpoint_model  SaveFormat=Structure With Time  SampleTime=Tc
  To Workspace4 : ToWorkspace  VariableName=rollrate_setpoint_model  SaveFormat=Structure With Time  SampleTime=Tq
  To Workspace5 : ToWorkspace  VariableName=y_command_model  SaveFormat=Structure With Time  SampleTime=Tq
  To Workspace6 : ToWorkspace  VariableName=z_command_model  SaveFormat=Structure With Time  SampleTime=Tc
  To Workspace7 : ToWorkspace  VariableName=yawrate_setpoint_model  SaveFormat=Structure With Time  SampleTime=Tc
  To Workspace8 : ToWorkspace  VariableName=yaw_command_model  SaveFormat=Structure With Time  SampleTime=Tq
  To Workspace9 : ToWorkspace  VariableName=x_position_model  SaveFormat=Structure With Time  SampleTime=Tc
  X PID Controller : Subsystem
  X Velocity PID Controller : Subsystem
  Y PID Controller : Subsystem
  Y PID Controller1 : Subsystem
  Y PID Controller2 : Subsystem
  Y Velocity PID Controller : Subsystem
  Yaw Controller Input : Subsystem  Variant=on
  Yaw PID Controller : Subsystem
  Yaw Rate Controller Input : Subsystem  Variant=on
  Yaw Rate PID Controller : Subsystem
  Z PID Controller : Subsystem
  height_controlled : Outport
  y_controlled : Outport  Port=2
  x_controlled : Outport  Port=3
  yaw_controlled : Outport  Port=4
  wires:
  pitch_rate/1 -> Pitch Rate Controller Input/2(pitchrate_model), Scope6/1, Sum4/2
  z_setpoint/1 -> Sum7/1
  x_position/1 -> Sum5/2, Latitude Controller Input/2(x_position_model), Scope4/1, To Workspace9/1, Y PID Controller2/2(x_pos)
  Pitch PID Controller/1(pitchrate_setpoint) -> Sum4/1, To Workspace1/1
  pitch/1 -> Pitch Controller Input/2(pitch_angle_model), Gain/1, Sum3/2
  Gain/1 -> Scope9/1
  Yaw Rate PID Controller/1(yaw_motor_command) -> To Workspace8/1, Saturation/1
  Pitch Rate PID Controller/1(x_motor_command) -> Saturation1/1, To Workspace2/1
  x_setpoint/1 -> Sum5/1
  roll_rate/1 -> Roll Rate Controller Input/2(rollrate_model), Scope11/1, Sum10/2
  Roll PID Controller/1(rollrate_setpoint) -> Sum10/1, To Workspace4/1
  roll/1 -> Roll Controller Input/2(roll_angle_model), Gain2/1, Sum9/2
  Gain2/1 -> Scope13/1
  y_setpoint/1 -> Sum11/1
  yaw/1 -> Yaw Controller Input/2(yaw_angle_model), Scope3/1, To Workspace10/1, Sum1/2
  yaw_setpoint/1 -> Sum1/1
  yaw_rate/1 -> Gain1/1, Yaw Rate Controller Input/2(yawrate_model), Sum2/2
  Gain1/1 -> Scope1/1
  Yaw PID Controller/1(yawrate_setpoint) -> Sum2/1, To Workspace7/1
  z_position/1 -> Altitude Controller Input/2(z_position_model), To Workspace12/1, Scope2/1, Sum7/2
  Sum1/1 -> Yaw Controller Input/1(yaw_error_model)
  Sum2/1 -> Yaw Rate Controller Input/1(yawrate_error_model)
  Sum5/1 -> Latitude Controller Input/1(x_error_model), Y PID Controller2/1(x_error)
  Sum3/1 -> Pitch Controller Input/1(pitch_error_model)
  Sum4/1 -> Pitch Rate Controller Input/1(pitchrate_error_model)
  Sum9/1 -> Roll Controller Input/1(roll_error_model)
  Sum10/1 -> Roll Rate Controller Input/1(rollrate_error_model)
  Sum7/1 -> Altitude Controller Input/1(z_error_model)
  Roll Rate PID Controller/1(y_motor_command) -> To Workspace5/1, Saturation2/1
  Saturation3/1 -> height_controlled/1
  Saturation2/1 -> y_controlled/1
  Saturation1/1 -> x_controlled/1
  Saturation/1 -> yaw_controlled/1
  Longitude Controller Input/2(y_position) -> Y PID Controller/2(y_pos)
  Longitude Controller Input/1(y_error) -> Y PID Controller/1(y_error)
  y_position/1 -> Longitude Controller Input/2(y_position_model), Y PID Controller1/2(y_pos), To Workspace11/1, Scope12/1, Sum11/2
  Latitude Controller Input/1(x_error) -> X PID Controller/1(x_error)
  Latitude Controller Input/2(x_position) -> X PID Controller/2(x_pos)
  Yaw Controller Input/1(yaw_error) -> Yaw PID Controller/1(yaw_error)
  Yaw Controller Input/2(yaw_angle) -> Yaw PID Controller/2(yaw_angle)
  Altitude Controller Input/1(z_error) -> Z PID Controller/1(z_error)
  Altitude Controller Input/2(z_position) -> Z PID Controller/2(z_pos)
  Pitch Controller Input/1(pitch_error) -> Pitch PID Controller/1(pitch_error)
  Pitch Controller Input/2(pitch_angle) -> Pitch PID Controller/2(pitch_angle)
  Yaw Rate Controller Input/1(yawrate_error) -> Yaw Rate PID Controller/1(yawrate_error)
  Yaw Rate Controller Input/2(yawrate) -> Yaw Rate PID Controller/2(yawrate)
  Pitch Rate Controller Input/1(pitchrate_error) -> Pitch Rate PID Controller/1(pitchrate_error)
  Pitch Rate Controller Input/2(pitchrate) -> Pitch Rate PID Controller/2(pitchrate)
  Roll Controller Input/1(roll_error) -> Roll PID Controller/1(roll_error)
  Roll Controller Input/2(roll_angle) -> Roll PID Controller/2(roll_angle)
  Roll Rate Controller Input/1(rollrate_error) -> Roll Rate PID Controller/1(rollrate_error)
  Roll Rate Controller Input/2(rollrate) -> Roll Rate PID Controller/2(rollrate)
  Sum11/1 -> Longitude Controller Input/1(y_error_model), Y PID Controller1/1(y_error)
  Y PID Controller/1(roll_setpoint) -> To Workspace13/1, Sum6/1
  Y PID Controller1/1(y_vel_setpoint) -> Longitude Controller Input1/2(y_vel_model), Sum6/2
  Sum6/1 -> Longitude Controller Input1/1(y_vel_error_model)
  Longitude Controller Input1/1(y_vel_error) -> Y Velocity PID Controller/1(y_error)
  Longitude Controller Input1/2(y_vel) -> Y Velocity PID Controller/2(y_pos)
  Y Velocity PID Controller/1(roll_setpoint) -> To Workspace3/1, Sum9/1
  X PID Controller/1(pitch_setpoint) -> To Workspace14/1, Sum8/1
  Y PID Controller2/1(x_vel_setpoint) -> Longitude Controller Input2/2(x_vel_model), Sum8/2
  Sum8/1 -> Longitude Controller Input2/1(x_vel_error_model)
  Longitude Controller Input2/1(x_vel_error) -> X Velocity PID Controller/1(x_vel_error)
  Longitude Controller Input2/2(x_vel) -> X Velocity PID Controller/2(x_vel)
  X Velocity PID Controller/1(pitch_setpoint) -> To Workspace/1, Sum3/1
  Z PID Controller/1(z_motor_command) -> To Workspace6/1, Saturation3/1

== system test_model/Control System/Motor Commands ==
  note: 1) Add Subsystem or Model blocks as valid variant choices. 2) You cannot connect blocks at this level. At simulation, connectivity is automatically determined, based on the active variant and port name matching.
  z_command_model : Inport
  Feedback : Subsystem  VariantControl=logAnalysisToggle==0
  Motor Command : Subsystem  VariantControl=logAnalysisToggle==1
  z_command : Outport

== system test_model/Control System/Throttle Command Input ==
  note: 1) Add Subsystem or Model blocks as valid variant choices. 2) You cannot connect blocks at this level. At simulation, connectivity is automatically determined, based on the active variant and port name matching.
  Auto Takeoff : Subsystem  VariantControl=logAnalysisToggle==1
  height_controlled_o : Subsystem  VariantControl=logAnalysisToggle==0
  z_command : Outport

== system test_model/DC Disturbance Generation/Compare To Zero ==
  u : Inport
  Compare : RelationalOperator  Operator=~=  OutDataTypeStr=fixdt(0, 8)
  Constant : Constant  DisableCoverage=on  Value=0  OutDataTypeStr=Inherit: Inherit via back propagation  PreserveConstantTs=on
  y : Outport
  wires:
  Constant/1 -> Compare/2
  u/1 -> Compare/1
  Compare/1 -> y/1

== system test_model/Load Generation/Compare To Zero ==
  u : Inport
  Compare : RelationalOperator  Operator=~=  OutDataTypeStr=fixdt(0, 8)
  Constant : Constant  DisableCoverage=on  Value=0  OutDataTypeStr=Inherit: Inherit via back propagation  PreserveConstantTs=on
  y : Outport
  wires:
  Constant/1 -> Compare/2
  u/1 -> Compare/1
  Compare/1 -> y/1

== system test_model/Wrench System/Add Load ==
  m_0 : Inport
  J_0 : Inport  Port=2
  r_oc_0 : Inport  Port=3
  m_l : Inport  Port=4
  J_l : Inport  Port=5
  r_ol : Inport  Port=6
  Add Load to Quadrotor : MATLAB Function  TreatAsAtomicUnit=on
  m : Outport
  J : Outport  Port=2
  r_oc : Outport  Port=3
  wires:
  r_ol/1 -> Add Load to Quadrotor/6(r_ol)
  Add Load to Quadrotor/3(r_oc) -> r_oc/1
  J_l/1 -> Add Load to Quadrotor/5(J_l)
  m_l/1 -> Add Load to Quadrotor/4(m_l)
  Add Load to Quadrotor/2(J) -> J/1
  r_oc_0/1 -> Add Load to Quadrotor/3(r_oc_0)
  J_0/1 -> Add Load to Quadrotor/2(J_0)
  Add Load to Quadrotor/1(m) -> m/1
  m_0/1 -> Add Load to Quadrotor/1(m_0)

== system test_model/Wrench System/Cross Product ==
  note: Cross product of two 3x1 vectors a=[a1 a2 a3], b=[b1 b2 b3]: y = a x b = (a2b3 - a3b2)i + (a3b1 - a1b3)j + (a1b2 - a2b1)k
  a : Inport
  b : Inport  Port=2
  Add3 : Sum  Inputs=+-
  Demux2 : Demux  Outputs=2
  Element product : Product
  a elements : Selector  InputPortWidth=3  IndexOptions=Index vector (dialog)  Indices=[2 3 1 3 1 2]  OutputSizes=1
  b elements : Selector  InputPortWidth=3  IndexOptions=Index vector (dialog)  Indices=[3 1 2 2 3 1]  OutputSizes=1
  y : Outport
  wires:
  Add3/1 -> y/1
  Demux2/2 -> Add3/2
  Demux2/1 -> Add3/1
  Element product/1 -> Demux2/1
  a/1 -> a elements/1
  b/1 -> b elements/1
  b elements/1 -> Element product/2
  a elements/1 -> Element product/1

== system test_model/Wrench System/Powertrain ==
  P : Inport
  Lambda : Inport  Port=2
  8 Inch Rotor System : Subsystem
  Battery : Subsystem
  ESC-BLDC Motor System : Subsystem
  W_r : Outport
  M : Outport  Port=2
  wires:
  8 Inch Rotor System/1(W_r) -> W_r/1
  Lambda/1 -> 8 Inch Rotor System/2(Lambda)
  P/1 -> ESC-BLDC Motor System/1(P)
  Battery/1(V) -> ESC-BLDC Motor System/2(V_b)
  ESC-BLDC Motor System/1(M) -> 8 Inch Rotor System/1(M), M/1

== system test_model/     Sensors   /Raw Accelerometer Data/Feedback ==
  raw_accel_model : Inport
  raw_accel : Outport
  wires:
  raw_accel_model/1 -> raw_accel/1

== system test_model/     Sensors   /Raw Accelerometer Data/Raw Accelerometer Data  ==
  From Workspace5 : FromWorkspace  VariableName=raw_accel_data  SampleTime=Tq
  raw_accel : Outport
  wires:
  From Workspace5/1 -> raw_accel/1

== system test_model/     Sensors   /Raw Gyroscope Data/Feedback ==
  raw_gyro_model : Inport
  raw_gyro : Outport
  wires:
  raw_gyro_model/1 -> raw_gyro/1

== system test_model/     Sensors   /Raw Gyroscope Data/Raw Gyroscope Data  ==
  From Workspace5 : FromWorkspace  VariableName=raw_gyro_data  SampleTime=Tq
  raw_gyro : Outport
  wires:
  From Workspace5/1 -> raw_gyro/1

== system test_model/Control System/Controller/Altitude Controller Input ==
  note: 1) Add Subsystem or Model blocks as valid variant choices. 2) You cannot connect blocks at this level. At simulation, connectivity is automatically determined, based on the active variant and port name matching.
  z_error_model : Inport
  z_position_model : Inport  Port=2
  Feedback : Subsystem  VariantControl=logAnalysisToggle==0
  z error : Subsystem  VariantControl=logAnalysisToggle==1
  z_error : Outport
  z_position : Outport  Port=2

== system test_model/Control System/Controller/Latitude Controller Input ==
  note: 1) Add Subsystem or Model blocks as valid variant choices. 2) You cannot connect blocks at this level. At simulation, connectivity is automatically determined, based on the active variant and port name matching.
  x_error_model : Inport
  x_position_model : Inport  Port=2
  Feedback : Subsystem  VariantControl=logAnalysisToggle==0
  log : Subsystem  VariantControl=logAnalysisToggle==1
  x_error : Outport
  x_position : Outport  Port=2

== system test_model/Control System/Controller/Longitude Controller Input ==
  note: 1) Add Subsystem or Model blocks as valid variant choices. 2) You cannot connect blocks at this level. At simulation, connectivity is automatically determined, based on the active variant and port name matching.
  y_error_model : Inport
  y_position_model : Inport  Port=2
  Feedback : Subsystem  VariantControl=logAnalysisToggle==0
  y error : Subsystem  VariantControl=logAnalysisToggle==1
  y_error : Outport
  y_position : Outport  Port=2

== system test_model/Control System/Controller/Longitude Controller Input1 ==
  note: 1) Add Subsystem or Model blocks as valid variant choices. 2) You cannot connect blocks at this level. At simulation, connectivity is automatically determined, based on the active variant and port name matching.
  y_vel_error_model : Inport
  y_vel_model : Inport  Port=2
  Feedback : Subsystem  VariantControl=logAnalysisToggle==0
  y error : Subsystem  VariantControl=logAnalysisToggle==1
  y_vel_error : Outport
  y_vel : Outport  Port=2

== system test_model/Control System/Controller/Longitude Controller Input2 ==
  note: 1) Add Subsystem or Model blocks as valid variant choices. 2) You cannot connect blocks at this level. At simulation, connectivity is automatically determined, based on the active variant and port name matching.
  x_vel_error_model : Inport
  x_vel_model : Inport  Port=2
  Feedback : Subsystem  VariantControl=logAnalysisToggle==0
  y error : Subsystem  VariantControl=logAnalysisToggle==1
  x_vel_error : Outport
  x_vel : Outport  Port=2

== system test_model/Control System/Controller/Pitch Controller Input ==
  note: 1) Add Subsystem or Model blocks as valid variant choices. 2) You cannot connect blocks at this level. At simulation, connectivity is automatically determined, based on the active variant and port name matching.
  pitch_error_model : Inport
  pitch_angle_model : Inport  Port=2
  Feedback : Subsystem  VariantControl=logAnalysisToggle==0
  pitch error : Subsystem  VariantControl=logAnalysisToggle==1
  pitch_error : Outport
  pitch_angle : Outport  Port=2

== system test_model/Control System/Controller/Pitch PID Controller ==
  pitch_error : Inport
  pitch_angle : Inport  Port=2
  Add : Sum  Inputs=+-
  Discrete D Controller : Derivative/Discrete D Controller  Kd=Kd  a=a
  Discrete PI Controller : simulink/Continuous/PID Controller  Controller=PI  TimeDomain=Discrete-time  SampleTime=Ts  IntegratorMethod=Forward Euler  FilterMethod=Forward Euler  Form=Parallel  UseFilter=on  ControllerParametersSource=internal  P=Kp  I=Ki  D=0  N=100  InitialConditionSource=internal  InitialConditionForIntegrator=0  InitialConditionForFilter=0  ExternalReset=none  LimitOutput=off  UpperSaturationLimit=inf  LowerSaturationLimit=-inf  LinearizeAsGain=off  AntiWindupMode=none  Kb=1  TrackingMode=off  Kt=1  PParamMin=[]  PParamMax=[]  IParamMin=[]  IParamMax=[]  DParamMin=[]  DParamMax=[]  NParamMin=[]  NParamMax=[]  KbParamMin=[]  KbParamMax=[]  KtParamMin=[]  KtParamMax=[]  POutMin=[]  POutMax=[]  IOutMin=[]  IOutMax=[]  DOutMin=[]  DOutMax=[]  NOutMin=[]  NOutMax=[]  KbOutMin=[]  KbOutMax=[]  KtOutMin=[]  KtOutMax=[]  IntegratorOutMin=[]  IntegratorOutMax=[]  FilterOutMin=[]  FilterOutMax=[]  SumOutMin=[]  SumOutMax=[]  SumI1OutMin=[]  SumI1OutMax=[]  SumI2OutMin=[]  SumI2OutMax=[]  SumI3OutMin=[]  SumI3OutMax=[]  SumDOutMin=[]  SumDOutMax=[]  SaturationOutMin=[]  SaturationOutMax=[]  IntegratorContinuousStateAttributes=''  IntegratorStateMustResolveToSignalObject=off  IntegratorRTWStateStorageClass=Auto  FilterContinuousStateAttributes=''  FilterStateMustResolveToSignalObject=off  FilterRTWStateStorageClass=Auto  DifferentiatorICPrevScaledInput=0  DifferentiatorOutMin=[]  DifferentiatorOutMax=[]
  pitchrate_setpoint : Outport
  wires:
  pitch_angle/1 -> Discrete D Controller/1
  pitch_error/1 -> Discrete PI Controller/1
  Discrete PI Controller/1 -> Add/1
  Discrete D Controller/1 -> Add/2
  Add/1 -> pitchrate_setpoint/1
